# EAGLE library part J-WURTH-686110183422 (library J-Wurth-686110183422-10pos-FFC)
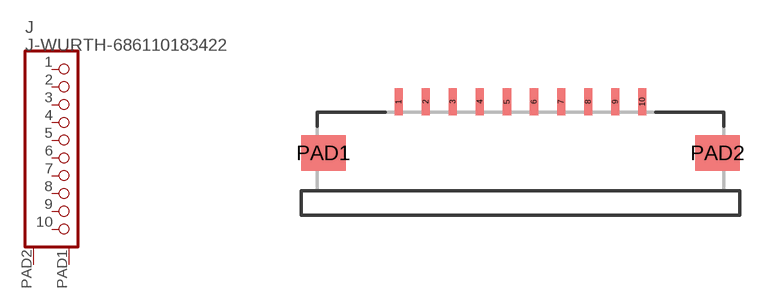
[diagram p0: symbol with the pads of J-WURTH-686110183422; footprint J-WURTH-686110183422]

Designator prefix J

## J-WURTH-686110183422  [J-WURTH-686110183422]
1  1  pas
2  2  pas
3  3  pas
4  4  pas
5  5  pas
6  6  pas
7  7  pas
8  8  pas
9  9  pas
10  10  pas
PAD1  PAD1  pas
PAD2  PAD2  pas

## Footprint J-WURTH-686110183422 (pad centres in mm)
smd 0.3 x 1: 1 -4.5,1.9; 2 -3.5,1.9; 3 -2.5,1.9; 4 -1.5,1.9; 5 -0.5,1.9; 6 0.5,1.9; 7 1.5,1.9; 8 2.5,1.9; 9 3.5,1.9; 10 4.5,1.9
smd 1.65 x 1.3: PAD1 -7.28,0; PAD2 7.28,0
